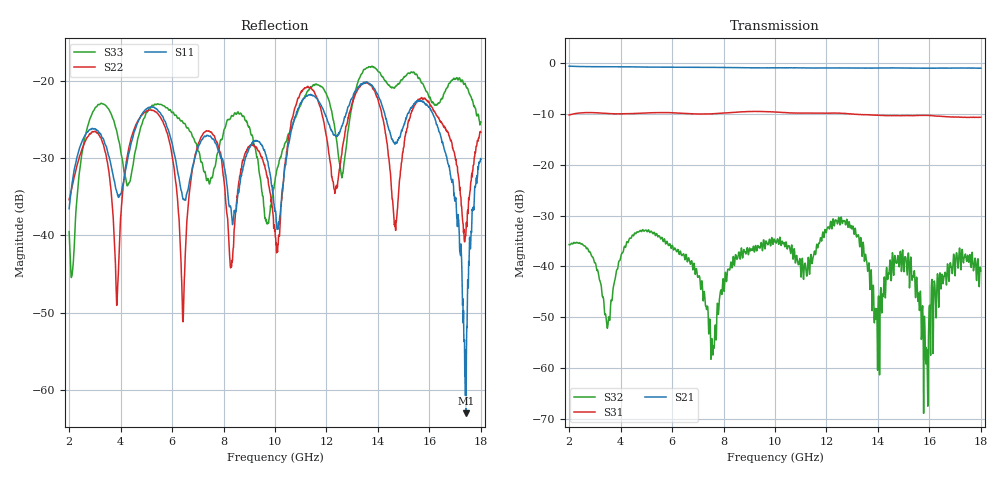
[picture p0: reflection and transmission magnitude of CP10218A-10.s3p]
! Amtery
! Email: info@amtery.com
! Phone: 886-2-2883-7839
! Model Number: CP10218A-10
! 3-port S-parameter measurement data for Directional Coupler
! Frequency Range: 2 GHz to 18 GHz
! Port 1: Input
! Port 2: Output
! Port 3: Coupled
# hz S db R 50
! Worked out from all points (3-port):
!   1281 points, 2 GHz to 18 GHz, reference 50 ohm
!   strongest paths, dB at 2 GHz, 6 GHz, 10 GHz, 14 GHz, 18 GHz:
!     S21: -0.6, -0.8, -0.9, -1.0, -1.0
!     S31: -10.2, -9.8, -9.6, -10.2, -10.7
!     S32: -35.7, -35.9, -35.1, -49.2, -40.9
!   lowest |S11| = -63.0 dB at 17.43 GHz (marker M1), VSWR 1.00, Z = 50 - j0.053 ohm
!   |S11| at or under -10 dB: start of sweep to end of sweep
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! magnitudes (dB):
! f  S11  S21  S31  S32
! 2 GHz  -36.5  -0.6  -10.2  -35.7
! 3.862 GHz  -34.5  -0.7  -10.0  -40.6
! 5.388 GHz  -23.6  -0.8  -9.7  -33.6
! 6.425 GHz  -35.3  -0.8  -9.9  -37.6
! 7.575 GHz  -27.5  -0.8  -10.0  -57.0
! 10 GHz  -36.9  -0.9  -9.6  -35.1
! 11.1 GHz  -22.3  -0.9  -9.8  -42.4
! 15.74 GHz  -22.6  -1.0  -10.3  -47.7
! 17.43 GHz  -63.0  -1.0  -10.7  -38.2
! 18 GHz  -30.1  -1.0  -10.7  -40.9
